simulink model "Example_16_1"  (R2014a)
settings: Solver=ode45  StartTime=0.0  StopTime=10.0  RelTol=1e-3

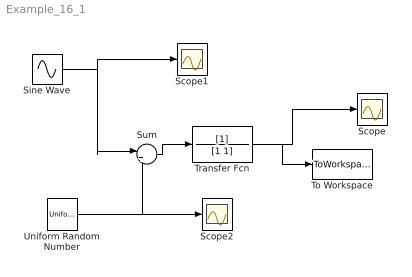
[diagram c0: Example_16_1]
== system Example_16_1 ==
  Scope : Scope
  Scope1 : Scope
  Scope2 : Scope
  Sine Wave : Sin  Amplitude=5  Frequency=2  SampleTime=0
  Sum : Sum  Inputs=|++
  To Workspace : ToWorkspace  VariableName=simout  SaveFormat=Timeseries  SampleTime=-1
  Transfer Fcn : TransferFcn  Denominator=[1 1]
  Uniform Random Number : UniformRandomNumber  SampleTime=0.1
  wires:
  Sine Wave/1 -> Sum/1, Scope1/1
  Uniform Random Number/1 -> Sum/2, Scope2/1
  Transfer Fcn/1 -> To Workspace/1, Scope/1
  Sum/1 -> Transfer Fcn/1
